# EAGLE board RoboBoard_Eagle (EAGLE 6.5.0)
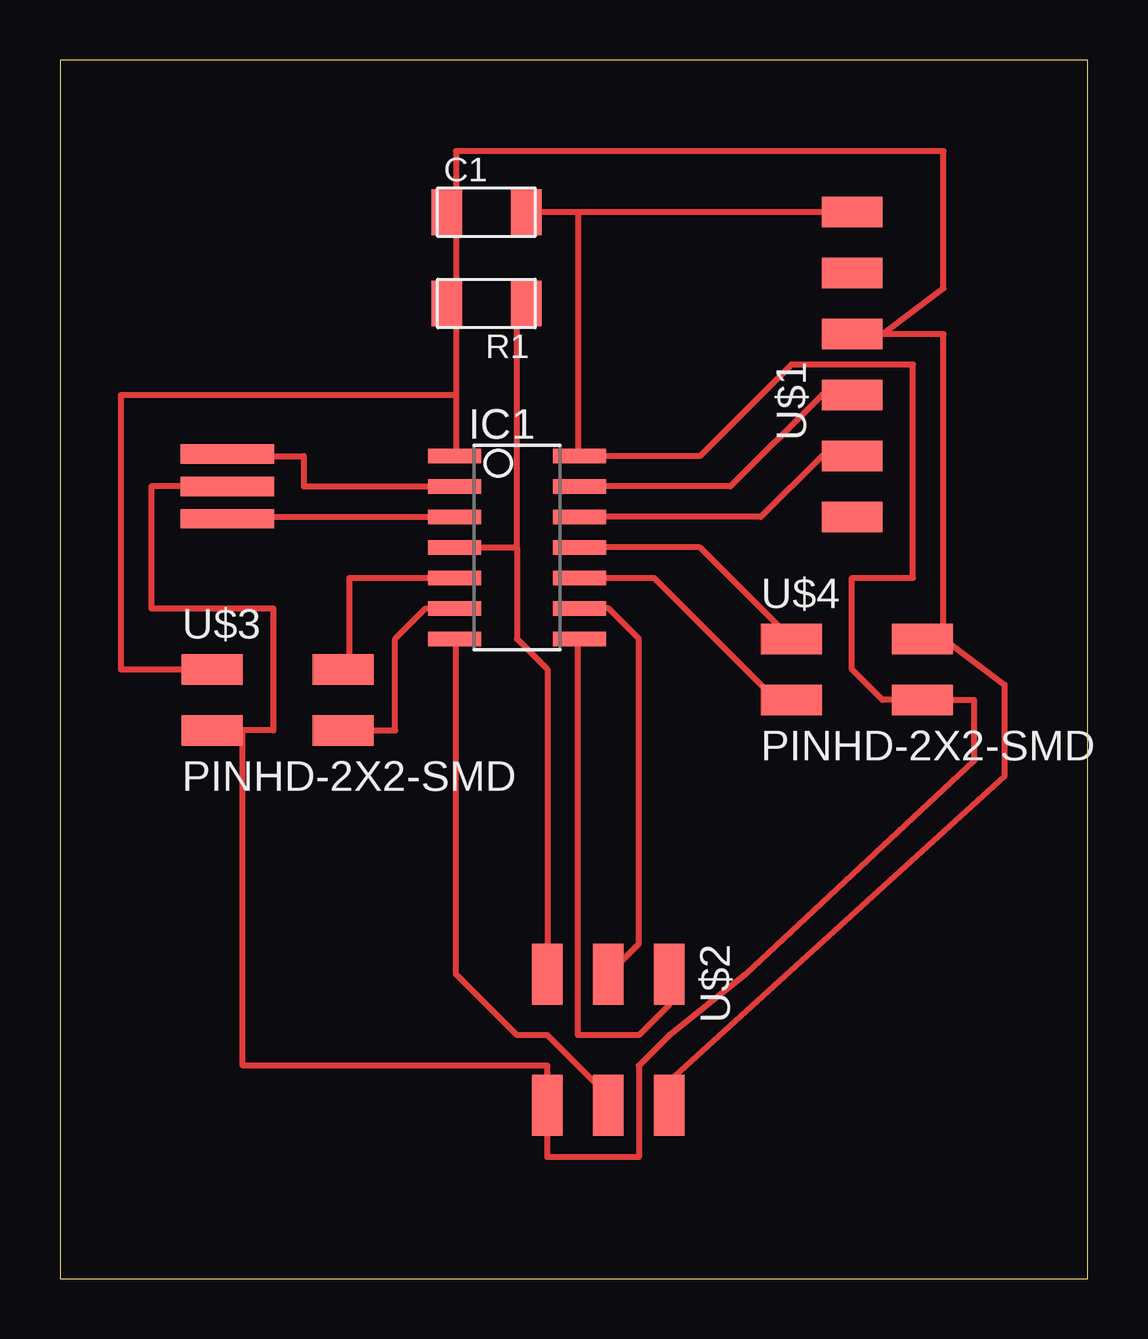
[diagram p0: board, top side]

Size 42.85 x 50.79 mm. Coordinates in mm from the lower left corner, seen from the top.
Outline: 0,0 42.85,0 42.85,50.79 0,50.79 0,0
Copper layers (1*16): Top 0.035mm / dielectric 1.5mm / Bottom 0.035mm
Design rules "default *": minimum track width 10mil, minimum drill 24mil, track to track 15mil, track to pad 15mil, pad to pad 15mil, via to via 15mil, smd to smd 15mil, copper to edge 40mil, drill to drill 8mil, minimum pad ring 10mil, minimum via ring 8mil, stop-mask expansion 4mil, vias tented up to drill 0mil, thermal gap 10mil

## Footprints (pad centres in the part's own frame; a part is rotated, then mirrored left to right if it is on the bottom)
EFOBM = smd 0.8 x 3.9: 1 -1.35,0; 2 0,0; 3 1.35,0
C1206FAB = smd 1.27 x 1.905: 1 -1.651,0; 2 1.651,0
SOIC14 = smd 0.61 x 2.21: 1 -3.81,-2.603; 2 -2.54,-2.603; 3 -1.27,-2.603; 4 0,-2.603; 5 1.27,-2.603; 6 2.54,-2.603; 7 3.81,-2.603; 8 3.81,2.603; 9 2.54,2.603; 10 1.27,2.603; 11 0,2.603; 12 -1.27,2.603; 13 -2.54,2.603; 14 -3.81,2.603
R1206FAB = smd 1.27 x 1.905: 1 -1.651,0; 2 1.651,0
1X06SMD = smd 2.54 x 1.27: 1 0,6.35; 2 0,3.81; 3 0,1.27; 4 0,-1.27; 5 0,-3.81; 6 0,-6.35
2X03SMD = smd 2.54 x 1.27: 1 -2.54,2.54; 2 2.92,2.54; 3 -2.54,0; 4 2.92,0; 5 -2.54,-2.54; 6 2.92,-2.54
2X02SMD = smd 2.54 x 1.27: 1 -2.54,1.27; 2 2.92,1.27; 3 -2.54,-1.27; 4 2.92,-1.27

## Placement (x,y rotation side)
20MHZ  RESONATOR  [EFOBM]  6.99,33.02 270 top
C1  1uF  [C1206FAB]  17.78,44.45 0 top
IC1  ATTINY44-SSU  [SOIC14]  19.05,30.48 270 top
R1  10K  [R1206FAB]  17.78,40.64 180 top
U$1  FTDI-SMD-HEADER  [1X06SMD]  33.02,38.1 0 top
U$2  AVRISPSMD  [2X03SMD]  22.86,10.16 270 top
U$3  PINHD-2X2-SMD  [2X02SMD]  8.89,24.13 0 top
U$4  PINHD-2X2-SMD  [2X02SMD]  33.02,25.4 0 top

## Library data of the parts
20MHZ C1 IC1 R1 U$1-U$4 = fab

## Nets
20MHZ: 20MHZ.1 IC1.2
+5V: C1.1 IC1.1 R1.2 U$1.3 U$2.2 U$3.1 U$4.2
GND: 20MHZ.2 C1.2 IC1.14 U$1.1 U$2.6 U$3.3 U$4.4
MISO: IC1.8 U$2.1
MOSI: IC1.7 U$2.4
N$3: 20MHZ.3 IC1.3
PA2: IC1.11 U$4.1
PA3: IC1.10 U$4.3
PA7: IC1.6 U$3.4
PB2: IC1.5 U$3.2
RST: IC1.4 R1.1 U$2.5
RX: IC1.12 U$1.5
SCK: IC1.9 U$2.3
TX: IC1.13 U$1.4

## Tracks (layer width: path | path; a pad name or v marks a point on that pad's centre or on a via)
20MHZ
  Top 0.254: 16.51,33.02 IC1.2 10.16,33.02 10.16,34.29 6.35,34.29 20MHZ.1
+5V
  Top 0.254: 16.51,44.45 16.51,40.64 | 16.51,44.45 C1.1 | 16.51,40.64 16.51,36.83 | 16.51,36.83 16.51,34.29 IC1.1 | 16.51,40.64 R1.2 | U$3.1 2.54,25.4 2.54,36.83 16.51,36.83 | 36.83,26.67 39.37,24.77 39.37,20.95 25.4,8.26 U$2.2 | 34.29,39.37 36.83,39.37 36.83,26.67 | 34.29,39.37 U$1.3 | 36.83,26.67 U$4.2 | 34.29,39.37 36.83,41.27 36.83,46.99 16.51,46.99 16.51,44.45
GND
  Top 0.254: U$1.1 21.59,44.45 | 21.59,44.45 C1.2 19.05,44.45 | 21.59,44.45 21.59,34.29 IC1.14 26.67,34.29 30.48,38.1 35.56,38.1 35.56,29.21 33.02,29.21 33.02,25.4 34.29,24.13 U$4.4 38.1,24.13 38.1,21.59 28.57,12.7 25.4,10.16 24.13,8.89 24.13,5.08 20.32,5.08 U$2.6 20.32,8.89 7.62,8.89 7.62,22.86 | 7.62,22.86 U$3.3 | 7.62,22.86 8.89,22.86 8.89,27.94 3.81,27.94 3.81,33.02 20MHZ.2
MISO
  Top 0.254: IC1.8 21.59,26.67 21.59,10.16 24.13,10.16 25.4,11.43 U$2.1
MOSI
  Top 0.254: IC1.7 16.51,26.67 16.51,12.7 19.05,10.16 20.32,10.16 22.86,7.62 U$2.4
N$3
  Top 0.254: 16.51,31.75 IC1.3 6.35,31.75 20MHZ.3
PA2
  Top 0.254: U$4.1 26.67,30.48 IC1.11 21.59,30.48
PA3
  Top 0.254: 21.59,29.21 IC1.10 24.77,29.21 29.84,24.13 U$4.3 31.11,24.13
PA7
  Top 0.254: U$3.4 13.97,22.86 13.97,26.67 15.24,27.94 IC1.6 16.51,27.94
PB2
  Top 0.254: 16.51,29.21 IC1.5 12.06,29.21 12.06,25.4 U$3.2
RST
  Top 0.254: 19.05,30.48 19.05,40.64 R1.1 | IC1.4 19.05,30.48 | U$2.5 20.32,25.4 19.05,26.67 19.05,30.48
RX
  Top 0.254: U$1.5 31.75,34.29 29.21,31.75 IC1.12 21.59,31.75
SCK
  Top 0.254: U$2.3 24.13,13.97 24.13,26.67 22.86,27.94 IC1.9 21.59,27.94
TX
  Top 0.254: U$1.4 31.75,36.83 27.94,33.02 IC1.13 21.59,33.02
